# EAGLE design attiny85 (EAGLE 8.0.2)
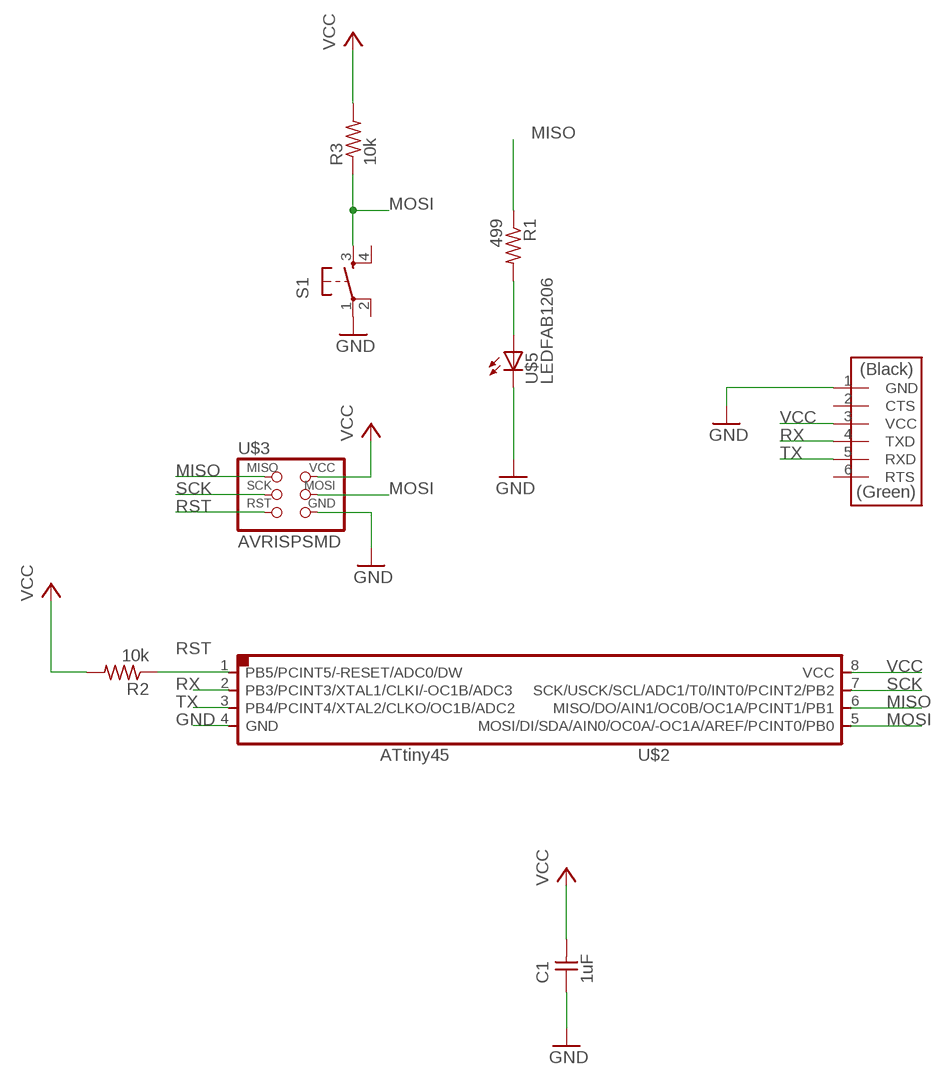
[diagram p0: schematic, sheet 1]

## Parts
C1  1uF  CAP-UNPOLARIZEDFAB  [C1206FAB]
R1  499  RES-US1206FAB  [R1206FAB]
R2  10k  RES-US1206FAB  [R1206FAB]
R3  10k  RES-US1206FAB  [R1206FAB]
S1  6MM_SWITCH6MM_SWITCH  [6MM_SWITCH]
U$2  ATTINY45SI  [SOIC8]
U$3  AVRISPSMD  [2X03SMD]
U$4  FTDI-SMD-HEADER  [1X06SMD]
U$5  LEDFAB1206  [LED1206FAB]

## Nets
GND: C1.1 S1.1(P) U$2.4(GND) U$3.6(GND) U$4.1(GND) U$5.2(C)
MISO: R1.1 U$2.6(MISO/DO/AIN1/OC0B/OC1A/PCINT1/PB1) U$3.1(MISO)
MOSI: R3.1 S1.3(S) U$2.5(MOSI/DI/SDA/AIN0/OC0A/-OC1A/AREF/PCINT0/PB0) U$3.4(MOSI)
N$6: R1.2 U$5.1(A)
RST: R2.1 U$2.1(PB5/PCINT5/-RESET/ADC0/DW) U$3.5(RST)
RX: U$2.2(PB3/PCINT3/XTAL1/CLKI/-OC1B/ADC3) U$4.4(TXD)
SCK: U$2.7(SCK/USCK/SCL/ADC1/T0/INT0/PCINT2/PB2) U$3.3(SCK)
TX: U$2.3(PB4/PCINT4/XTAL2/CLKO/OC1B/ADC2) U$4.5(RXD)
VCC: C1.2 R2.2 R3.2 U$2.8(VCC) U$3.2(VCC) U$4.3(VCC)
Unconnected: S1.2(P1) S1.4(S1) U$4.2(CTS) U$4.6(RTS)

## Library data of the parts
C1 = fab:CAP-UNPOLARIZED
R1-R3 = fab:RES-US: Resistor (US Symbol)
S1 = fab:6MM_SWITCH: OMRON SWITCH
U$2 = fab:ATTINY45
U$3 = fab:AVRISP
U$4 = fab:FTDI-SMD-HEADER
U$5 = fab:LED: LED

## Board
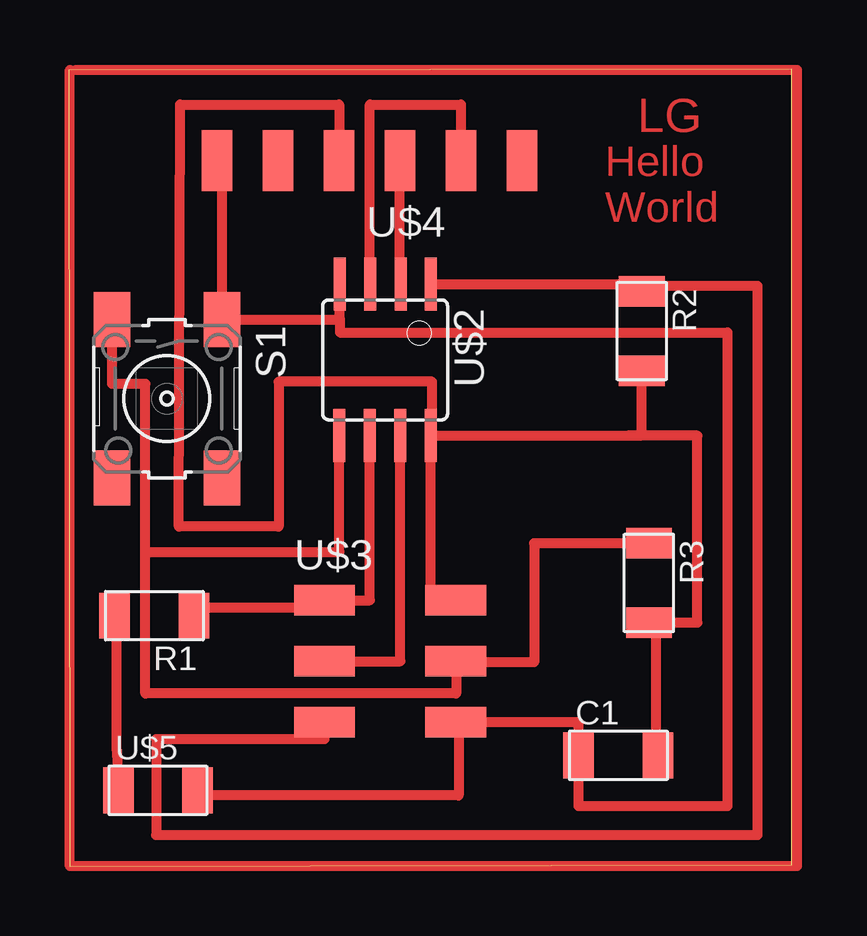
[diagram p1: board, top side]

Size 30.14 x 33.23 mm. Coordinates in mm from the lower left corner, seen from the top.
Outline: 0.05,0 30.14,0.05 30.14,33.23 0,33.18 0.05,0
Copper layers (1*16): Top 0.035mm / dielectric 1.5mm / Bottom 0.035mm
Design rules "default *": minimum track width 16mil, minimum drill 24mil, track to track 12mil, track to pad 12mil, pad to pad 8mil, via to via 8mil, smd to smd 8mil, copper to edge 40mil, drill to drill 8mil, minimum pad ring 10mil, minimum via ring 8mil, stop-mask expansion 4mil, vias tented up to drill 0mil, thermal gap 10mil

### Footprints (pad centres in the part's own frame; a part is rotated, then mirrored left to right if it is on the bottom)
C1206FAB = smd 1.27 x 1.905: 1 -1.651,0; 2 1.651,0
R1206FAB = smd 1.27 x 1.905: 1 -1.651,0; 2 1.651,0
6MM_SWITCH = smd 2.286 x 1.524: 1 -3.302,2.286; 2 3.302,2.286; 3 -3.302,-2.286; 4 3.302,-2.286
SOIC8 = smd 0.5 x 2.2: 1 -1.905,-3.154; 2 -0.645,-3.154; 3 0.625,-3.154; 4 1.895,-3.154; 5 1.905,3.154; 6 0.635,3.154; 7 -0.635,3.154; 8 -1.905,3.154
2X03SMD = smd 2.54 x 1.27: 1 -2.54,2.54; 2 2.92,2.54; 3 -2.54,0; 4 2.92,0; 5 -2.54,-2.54; 6 2.92,-2.54
1X06SMD = smd 2.54 x 1.27: 1 0,6.35; 2 0,3.81; 3 0,1.27; 4 0,-1.27; 5 0,-3.81; 6 0,-6.35
LED1206FAB = smd 1.27 x 1.905: 1 -1.651,0; 2 1.651,0

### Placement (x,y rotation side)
C1  22.9,4.62 0 top
R1  3.58,10.44 180 top
R2  23.88,22.3 270 top
R3  24.18,11.8 270 top
S1  4.1,19.48 270 top
U$2  13.19,21.11 180 top
U$3  13.21,8.54 0 top
U$4  12.54,29.41 90 top
U$5  3.73,3.16 0 top

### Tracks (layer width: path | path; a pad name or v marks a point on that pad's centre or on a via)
GND
  Top 0.406: 5.38,3.1 U$5.2 5.38,2.95 16.25,2.95 16.25,6 U$3.6 21.25,6 C1.1 21.25,2.5 27.45,2.5 27.45,22.25 11.3,22.25 11.3,22.79 | U$4.1 6.39,29.36 S1.1 11.3,22.79 | 11.29,22.79 U$2.4 11.3,22.79
MISO
  Top 0.406: R1.1 5.31,10.76 10.6,10.76 U$3.1 | 10.93,11.09 U$3.1 | U$3.1 12.55,11.08 U$2.6
MOSI
  Top 0.406: 24.14,13.4 R3.1 19.4,13.46 19.4,8.5 16.12,8.5 U$3.4 | 16.21,8.45 U$3.4 | 2.01,22.64 S1.3 1.81,20.1 3.2,20.1 3.2,13.1 | U$3.4 16.15,8.54 16.15,7.2 3.2,7.2 3.2,13.1 | 3.2,13.1 11.29,13.1 U$2.5
N$6
  Top 0.406: R1.2 2.01,10.43 2.01,4.81 U$5.1
N$7
  Top 0.406: 0.3,33.2 30.35,33.2 30.35,0 0.05,0 0.05,33.2
RST
  Top 0.406: 23.81,23.96 R2.1 23.88,24.2 24.35,24.2 | 24.35,24.2 28.7,24.2 28.7,1.3 3.65,1.3 3.65,5.3 10.66,5.3 U$3.5 | U$2.1 24.35,24.26 24.35,24.2
RX
  Top 0.406: U$2.2 13.81,24.26 U$4.4
SCK
  Top 0.406: U$3.3 13.82,8.54 U$2.7
TX
  Top 0.406: U$2.3 12.55,24.26 12.55,31.75 16.35,31.75 U$4.5
VCC
  Top 0.406: C1.2 24.47,4.81 24.47,10.1 R3.2 26.2,10.15 26.2,17.95 23.35,17.95 | U$2.8 23.35,17.95 | 23.35,17.95 23.88,17.95 R2.2 | U$2.8 15.15,17.95 15.15,20.2 8.75,20.2 8.75,14.15 4.6,14.15 4.65,31.75 11.27,31.75 U$4.3 | U$3.2 15.09,11.08 U$2.8

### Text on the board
Top: LG | Hello / World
